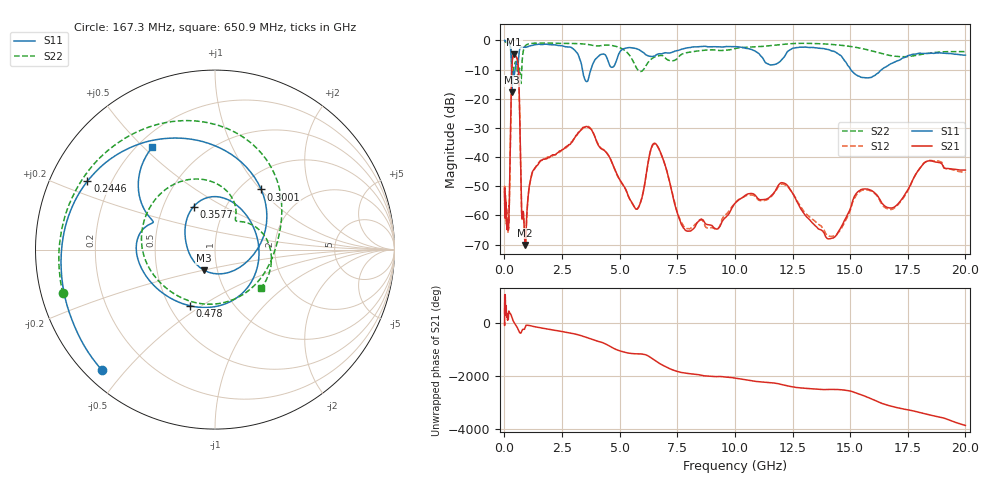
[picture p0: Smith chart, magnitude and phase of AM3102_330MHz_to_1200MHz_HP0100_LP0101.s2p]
! Date/Time: Tue, Sep 11, 2018 5:12 PM
! Network Analyzer: Agilent Technologies E8362B Rev: A.07.50.63
! Sweep from 0.010 to 20.000 GHz, 1601 Points, Sweep Type: LOG
! Power Supply: 4.949 V, 0.001 A
# Hz S DB R 50
!freq MagS11 AngS11 MagS21 AngS21 MagS12 AngS12 MagS22 AngS22
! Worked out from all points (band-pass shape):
!   1601 points, 10 MHz to 20 GHz, reference 50 ohm
!   highest |S21| = -4.71 dB at 424.4 MHz (marker M1); lowest = -70.1 dB at 899.1 MHz (marker M2)
!   |S21| within 3 dB of the highest: 335.7 MHz to 588.9 MHz (253.1 MHz wide, 54.8 % of centre)
!   lowest |S11| = -17.7 dB at 330 MHz (marker M3), VSWR 1.30, Z = 43.1 - j10.1 ohm
!   |S11| at or under -10 dB: 307.7 MHz to 463.5 MHz (155.8 MHz wide, 40.4 % of centre); 3.383 GHz to 3.756 GHz (372.5 MHz wide, 10.4 % of centre); 15.03 GHz to 16.37 GHz (1.346 GHz wide, 8.57 % of centre)
!   |S22| runs from -14.8 to -0.2 dB; largest |S21 - S12| = 0.0094
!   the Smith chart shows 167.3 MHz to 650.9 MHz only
!   S11 on the Smith chart (normalised r, x): 167.3 MHz: 0.05, -0.43; 244.6 MHz: 0.11, +0.25; 300.1 MHz: 1.24, +1.01; 357.7 MHz: 0.71, +0.37; 478 MHz: 0.63, -0.45; 650.9 MHz: 0.26, +0.53
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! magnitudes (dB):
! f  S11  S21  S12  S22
! 10 MHz  0.0  -52.6  -50.1  -0.2
! 35.55 MHz  0.0  -60.3  -58.4  -0.4
! 126.4 MHz  -0.4  -64.0  -61.8  -0.9
! 167.3 MHz  -0.7  -63.4  -64.4  -1.1
! 244.6 MHz  -1.9  -42.0  -42.1  -1.8
! 300.1 MHz  -7.5  -16.7  -16.8  -4.2
! 330 MHz  -17.7  -8.5  -8.5  -8.1
! 357.7 MHz  -11.5  -6.0  -6.1  -10.5
! 424.4 MHz  -12.1  -4.7  -4.7  -8.8
! 447.2 MHz  -10.8  -4.8  -4.8  -8.0
! 478 MHz  -9.3  -5.0  -5.1  -7.4
! 650.9 MHz  -3.5  -20.4  -20.4  -9.5
! 750.6 MHz  -2.3  -59.2  -59.4  -10.3
! 899.1 MHz  -2.4  -70.1  -70.3  -2.0
! 1.59 GHz  -1.4  -41.1  -41.2  -0.9
! 3.634 GHz  -13.6  -29.7  -29.5  -1.4
! 5.652 GHz  -2.6  -57.3  -57.4  -8.2
! 6.58 GHz  -5.0  -35.6  -35.7  -5.5
! 7.92 GHz  -2.6  -65.4  -64.5  -4.2
! 12.09 GHz  -6.1  -48.8  -49.2  -1.3
! 14.07 GHz  -3.2  -68.1  -67.1  -1.3
! 20 GHz  -5.0  -44.4  -45.3  -3.8
